(* Logix 5000 AddOnInstructionDefinition export; software revision 16.04 *)

ADD_ON_INSTRUCTION AMCI_ANG1E_Run_Blend_Move   (* revision 1.1, vendor AMCI, ExecuteEnableInFalse *)
// Revision note:
// Version 1.1 added the slot_axis number and the input parameters can now be tags or discrete values.
VAR_INPUT
   Axis_Status_bits : INT; {required}
   slot_axis_number : INT; {required}
   Direction_0_for_CW_1_for_CCW : BOOL; {required}
   Type_0_for_standard_1_for_indexed : BOOL;
END_VAR
VAR_IN_OUT
   AMCI_ANG1E_output_data : INT[10]; {required}
END_VAR
VAR_OUTPUT
   EN : BOOL; {visible}
   ER : BOOL; {visible}
END_VAR
VAR
   command_data_block : INT[10];
        [0]   // Command Bits MSW
        [1]   // Command Bits LSW
        [2]   // Upper Target Position
        [3]   // Lower Target Position
        [4]   // Upper Programmed Speed
        [5]   // Lower Programmed Speed
   index : INT;
END_VAR

ROUTINE EnableInFalse   (* ladder *)
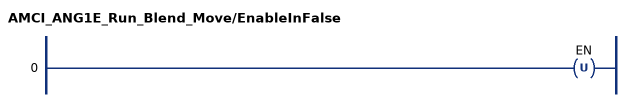
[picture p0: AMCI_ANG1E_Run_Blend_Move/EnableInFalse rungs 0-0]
   0: OTU(EN);
END_ROUTINE

ROUTINE Logic   (* ladder *)
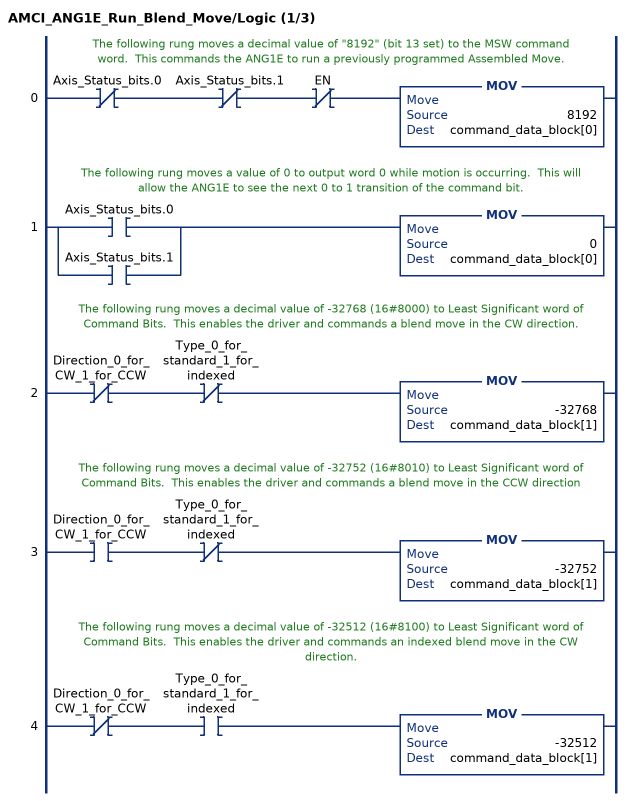
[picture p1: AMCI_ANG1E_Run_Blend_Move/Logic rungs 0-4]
   // The following rung moves a decimal value of "8192" (bit 13 set) to the MSW command word.  This commands the ANG1E to run a previously programmed Assembled Move.
   0: XIO(Axis_Status_bits.0)XIO(Axis_Status_bits.1)XIO(EN)MOV(8192,command_data_block[0]);
   // The following rung moves a value of 0 to output word 0 while motion is occurring.  This will allow the ANG1E to see the next 0 to 1 transition of the command bit.
   1: [XIC(Axis_Status_bits.0) ,XIC(Axis_Status_bits.1) ]MOV(0,command_data_block[0]);
   // The following rung moves a decimal value of -32768 (16#8000) to Least Significant word of Command Bits.  This enables the driver and commands a blend move in the CW direction.
   2: XIO(Direction_0_for_CW_1_for_CCW)XIO(Type_0_for_standard_1_for_indexed)MOV(-32768,command_data_block[1]);
   // The following rung moves a decimal value of -32752 (16#8010) to Least Significant word of Command Bits.  This enables the driver and commands a blend move in the CCW direction
   3: XIC(Direction_0_for_CW_1_for_CCW)XIO(Type_0_for_standard_1_for_indexed)MOV(-32752,command_data_block[1]);
   // The following rung moves a decimal value of -32512 (16#8100) to Least Significant word of Command Bits.  This enables the driver and commands an indexed blend move in the CW direction.
   4: XIO(Direction_0_for_CW_1_for_CCW)XIC(Type_0_for_standard_1_for_indexed)MOV(-32512,command_data_block[1]);
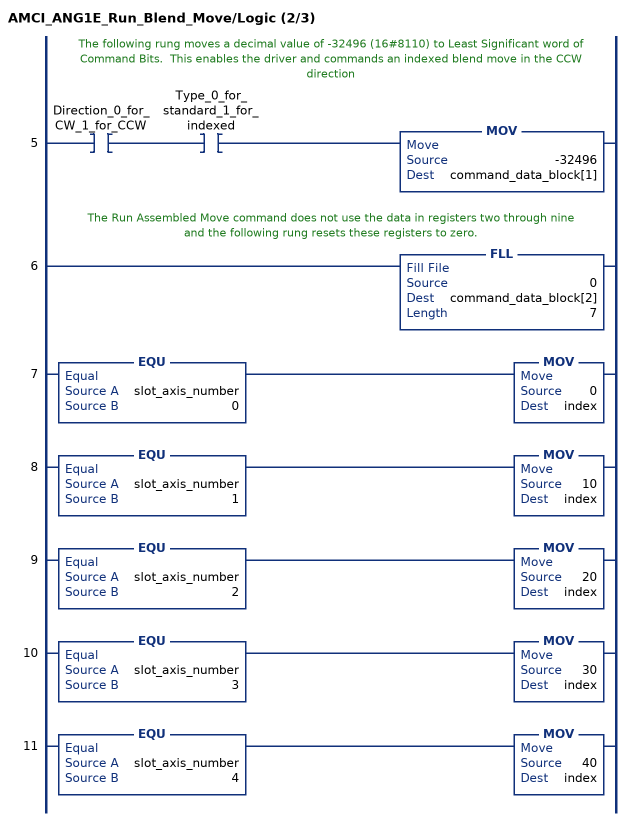
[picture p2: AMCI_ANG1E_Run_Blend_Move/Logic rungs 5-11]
   // The following rung moves a decimal value of -32496 (16#8110) to Least Significant word of Command Bits.  This enables the driver and commands an indexed blend move in the CCW direction
   5: XIC(Direction_0_for_CW_1_for_CCW)XIC(Type_0_for_standard_1_for_indexed)MOV(-32496,command_data_block[1]);
   // The Run Assembled Move command does not use the data in registers two through nine and the following rung resets these registers to zero.
   6: FLL(0,command_data_block[2],7);
   7: EQU(slot_axis_number,0)MOV(0,index);
   8: EQU(slot_axis_number,1)MOV(10,index);
   9: EQU(slot_axis_number,2)MOV(20,index);
   10: EQU(slot_axis_number,3)MOV(30,index);
   11: EQU(slot_axis_number,4)MOV(40,index);
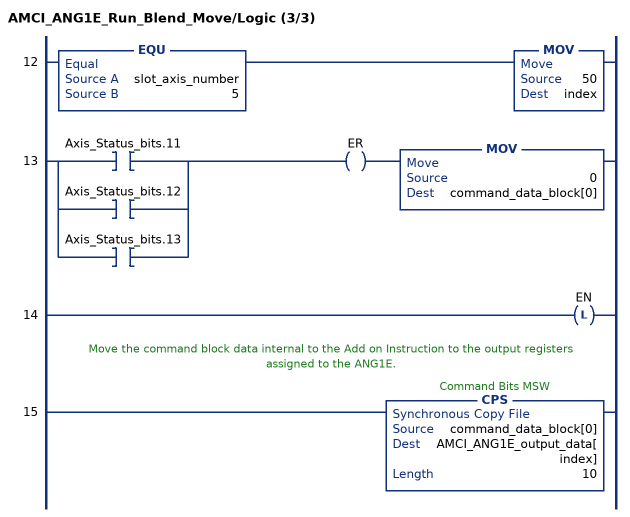
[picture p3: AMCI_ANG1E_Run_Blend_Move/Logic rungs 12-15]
   12: EQU(slot_axis_number,5)MOV(50,index);
   13: [XIC(Axis_Status_bits.11) ,XIC(Axis_Status_bits.12) ,XIC(Axis_Status_bits.13) ]OTE(ER)MOV(0,command_data_block[0]);
   14: OTL(EN);
   // Move the command block data internal to the Add on Instruction to the output registers assigned to the ANG1E.
   15: CPS(command_data_block[0],AMCI_ANG1E_output_data[index],10);
END_ROUTINE
END_ADD_ON_INSTRUCTION
